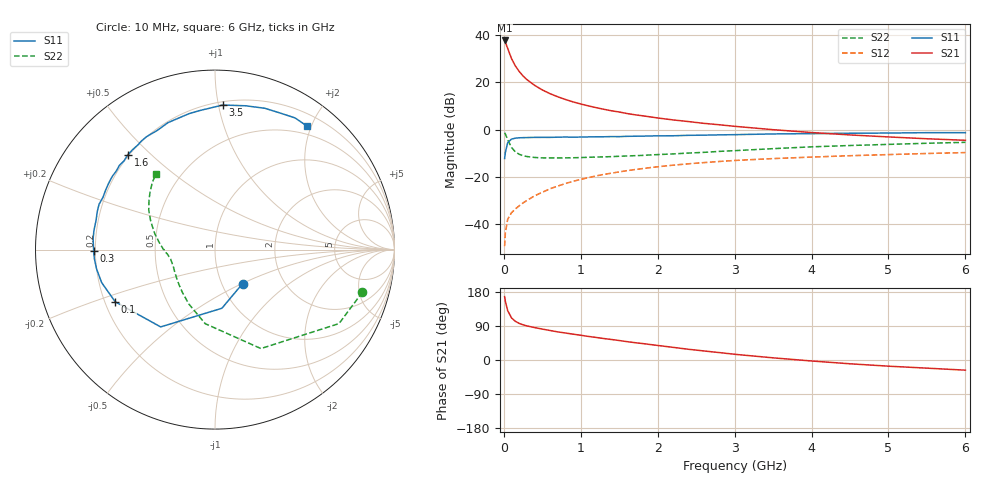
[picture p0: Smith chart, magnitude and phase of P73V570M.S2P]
! SIEMENS Small Signal Semiconductors
! BFP196
! Si NPN RF Bipolar Junction Transistor in SOT143
! VCE = 3.5 V  IC = 70 mA
! Common Emitter S-Parameters:  May  1996
# GHz  S  MA  R  50
!  f  S11  S21  S12  S22
! GHz  MAG  ANG  MAG  ANG  MAG  ANG  MAG  ANG
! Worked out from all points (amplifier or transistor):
!   36 points, 10 MHz to 6 GHz, reference 50 ohm
!   highest |S21| = 37.7 dB at 10 MHz (marker M1)
!   |S21| within 3 dB of that: start of sweep to 45.75 MHz
!   unconditionally stable (mu >= 1): 392.9 MHz to 4.418 GHz
!   at 250 MHz: K = 0.89, MSG = 26.9 dB, |S12| = -31.1 dB
!   at 1.4 GHz: K = 1.08, MAG = 11.4 dB, |S12| = -18.5 dB
!   at 6 GHz: K = 0.98, MSG = 2.6 dB, |S12| = -9.8 dB
!   S11 on the Smith chart (normalised r, x): 10 MHz: 1.25, -0.50; 100 MHz: 0.24, -0.23; 300 MHz: 0.19, -0.01; 1.6 GHz: 0.19, +0.43; 3.5 GHz: 0.22, +1.03; 6 GHz: 0.37, +1.94
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0.01  0.244 -51.0  76.8 167.2  0.0034 76.7  0.8549 -16.1
0.02  0.3291 -83.3  70.93 154.7  0.0065 71.1  0.8047 -30.8
0.05  0.5265 -125.1  52.03 130.2  0.0126 55.9  0.6079 -65.1
0.1  0.6275 -152.4  31.71 111.1  0.0174 50.5  0.4164 -97.5
0.15  0.6578 -163.8  22.16 102.0  0.0209 52.5  0.3363 -115.7
0.2  0.6686 -170.8  16.95 96.6  0.0243 55.5  0.2993 -127.5
0.25  0.6738 -175.5  13.57 92.8  0.028 57.7  0.2784 -136.5
0.3  0.6762 -179.3  11.39 90.0  0.0316 60.0  0.2681 -142.3
0.4  0.6818 174.8  8.617 85.5  0.0395 62.7  0.2564 -151.1
0.5  0.6828 170.9  6.888 81.6  0.047 64.3  0.2514 -156.7
0.6  0.6823 166.1  5.746 77.9  0.0557 64.7  0.2506 -160.6
0.7  0.6891 162.3  4.94 74.2  0.0635 64.6  0.2509 -163.3
0.8  0.6936 158.7  4.33 71.2  0.0719 63.6  0.2516 -165.7
0.9  0.6888 155.0  3.845 68.2  0.0802 63.3  0.2528 -167.9
1.1  0.6984 148.1  3.164 62.2  0.0959 61.5  0.2585 -170.8
1.6  0.718 132.5  2.183 48.5  0.1346 54.5  0.2761 -177.4
2.2  0.7378 115.9  1.599 33.4  0.176 45.6  0.3049 174.9
2.8  0.7711 100.8  1.262 19.6  0.2108 36.5  0.3447 165.7
3.5  0.8067 86.9  0.993 5.7  0.2428 26.4  0.3939 155.7
4.5  0.8349 70.6  0.769 -10.0  0.2794 14.3  0.4592 143.2
5.5  0.8586 58.7  0.638 -21.5  0.3112 3.6  0.5119 133.0
6  0.8582 53.1  0.592 -26.8  0.3254 -2.1  0.536 127.9
